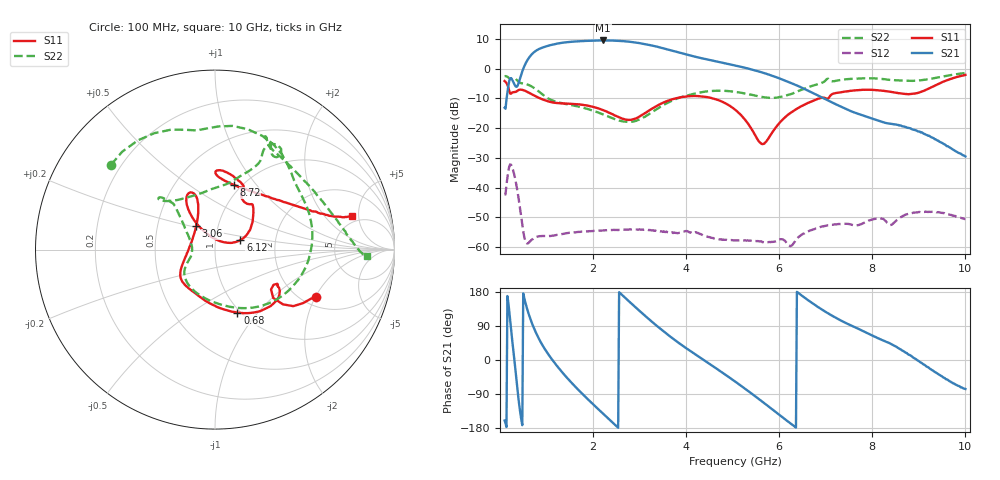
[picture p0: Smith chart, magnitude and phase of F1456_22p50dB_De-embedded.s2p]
! Integrated Device Technology
! Corporate Headquarters
! 6024 Silver Creek Valley Road
! San Jose, CA 95138  USA
! Phone:  1-408-284-8200
! Toll Free:  1-800-223-1366
! Webpage:  http://www.idt.com/
! Timing and RF Division
! 515 Groton Road, Suite 102
! Westford, MA 01886-6024
! Device:  F1456
! Description: 6-bit 0.5 dB Transmit Variable Gain Amplifier
! Frequency:  2100.0 -  2950.00 MHz
! Package:  6x6 mm Thin QFN Plastic Package: 28 pin
! State:  45
! Atten State:  22.5 dB
! Voltage:  +5.00 Volts
! Current:  216.961 mA
! Data:  The device was measured on a the F1455 evaluation board which has
!  individual transmission lines to the RF pins.  Data was collected
!  using a calibrated network analyzer.  The evaluation board was
!  de-embedded using a TRL calibration technique.
!  The reference plane is the edge of the package pin.
!  Pin  1 = CSb
!  Pin  2 = DATA
!  Pin  3 = CLK
!  Pin  4 = RSET
!  Pin  5 = GND
!  Pin  6 = RFIN  = Port 1
!  Pin  7 = GND
!  Pin  8 = NC
!  Pin  9 = NC
!  Pin 10 = NC
!  Pin 11 = NC
!  Pin 12 = NC
!  Pin 13 = NC
!  Pin 14 = /STBY
!  Pin 15 = GND
!  Pin 16 = RFOUT  = Port 2
!  Pin 17 = GND
!  Pin 18 = NC
!  Pin 19 = NC
!  Pin 20 = NC
!  Pin 21 = GND
!  Pin 22 = NC
!  Pin 23 = GND
!  Pin 24 = NC
!  Pin 25 = NC
!  Pin 26 = NC
!  Pin 27 = GND
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# GHz S dB R 50
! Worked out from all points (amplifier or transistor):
!   496 points, 100 MHz to 10 GHz, reference 50 ohm
!   highest |S21| = 9.5 dB at 2.22 GHz (marker M1)
!   |S21| within 3 dB of that: 824.2 MHz to 3.6 GHz (2.776 GHz wide, 125 % of centre)
!   unconditionally stable (mu >= 1): start of sweep to end of sweep
!   at 1.74 GHz: K = 84.36, MAG = 9.8 dB, |S12| = -54.8 dB
!   at 5.06 GHz: K = 272.75, MAG = 2.0 dB, |S12| = -57.7 dB
!   at 10 GHz: K = 554.66, MAG = -19.9 dB, |S12| = -50.6 dB
!   S11 on the Smith chart (normalised r, x): 100 MHz: 2.37, -2.01; 680 MHz: 0.97, -0.79; 3.06 GHz: 0.79, +0.21; 6.12 GHz: 1.32, +0.14; 8.72 GHz: 0.92, +0.77; 10 GHz: 4.18, +4.11
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0.1  -4.15 -24.9  -13.15 -159.8  -42.32 49.3  -2.53 140.8
0.24  -8.39 -31.0  -3.17 78.9  -32.36 -76.1  -3.41 94.4
0.32  -7.88 -30.0  -5.55 -11.2  -36.52 -153.5  -3.27 67.6
0.42  -7.07 -37.1  -3.87 -124.8  -45.70 140.7  -4.66 41.0
0.54  -7.42 -53.7  1.42 154.4  -57.74 132.8  -5.08 16.4
0.68  -8.56 -70.4  4.79 99.6  -57.58 143.6  -5.96 -15.7
0.86  -9.95 -88.6  6.78 50.6  -56.33 111.9  -7.99 -52.9
1.16  -11.41 -113.1  8.22 -5.3  -56.15 77.1  -10.87 -95.2
1.48  -11.75 -130.3  9.00 -52.3  -55.22 53.6  -12.08 -124.0
1.76  -12.10 -140.6  9.30 -88.1  -54.83 37.7  -13.01 -139.5
2.22  -13.95 -155.1  9.51 -142.2  -54.43 16.9  -15.42 -154.9
2.62  -16.75 178.0  9.32 172.1  -54.21 -0.1  -17.68 -170.4
3.06  -15.53 128.7  8.45 122.9  -54.12 -20.9  -16.66 159.6
3.4  -12.23 112.4  7.31 87.1  -54.58 -35.7  -13.32 142.5
4.1  -9.21 113.0  4.38 23.1  -55.10 -67.4  -8.69 133.1
5.06  -13.87 125.4  1.07 -57.5  -57.75 -116.4  -7.79 137.7
5.64  -25.38 69.0  -1.28 -110.3  -58.40 -158.5  -9.53 121.2
6.12  -16.42 20.5  -4.00 -156.1  -57.85 165.9  -9.10 87.0
6.7  -10.97 41.3  -7.99 150.9  -54.25 147.4  -5.82 64.4
8.36  -7.70 88.3  -18.46 45.0  -52.45 68.5  -3.74 62.4
8.72  -8.51 73.8  -19.61 19.2  -49.10 68.6  -4.04 50.2
10  -2.09 13.8  -29.53 -76.5  -50.60 -23.1  -1.46 -2.6
